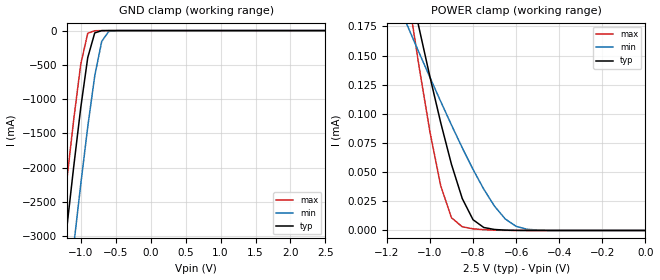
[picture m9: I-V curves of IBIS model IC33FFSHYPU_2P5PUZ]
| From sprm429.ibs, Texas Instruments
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|   Model IC33FFSHYPU_2P5PUZ
[Model]   IC33FFSHYPU_2P5PUZ
Model_type   Input
Polarity   Non-Inverting
Vinl =   0.7500V
Vinh =   1.7500V
C_comp   2.1510pF   2.1423pF   2.1675pF
[Temperature Range]   25.0000   0.1250k   -40.0000
[Voltage Range]   2.5000V   2.3000V   2.7000V
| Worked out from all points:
|   GND clamp passes 1 mA (typ) near -0.69 V on its own axis
|   POWER clamp passes 1 mA (typ) near -1.95 V on its own axis
[GND_clamp]
| voltage   I(typ)   I(min)   I(max)
-2.5V     -15.45A    -16.55A    -14.8A
-1.3V     -3.808A    -4.968A    -3.114A
-1.2V     -2.88A     -4.039A    -2.185A
-1.1V     -1.977A    -3.127A    -1.292A
-1V       -1.123A    -2.241A    -489.8mA
-900mV    -393.5mA   -1.402A    -39.29mA
-800mV    -34.07mA   -660.7mA   -2.405mA
-700mV    -1.067mA   -156.4mA   -232.2uA
-600mV    -42.99uA   -13.12mA   -13.27uA
-400mV    -95.57nA   -45.84uA   -11.77nA
2.5V      158.4pA    1.346nA    149.3pA
[POWER_clamp]
| voltage   I(typ)   I(min)   I(max)
-2.5V     1.522mA    806.3uA    2.102mA
-1.1V     216.2uA    173.8uA    200.1uA
-1.05V    173.4uA    152.4uA    140.2uA
-1V       131.9uA    131.4uA    84.68uA
-950mV    92.55uA    110.7uA    38.41uA
-900mV    56.73uA    90.48uA    10.93uA
-850mV    27.42uA    70.97uA    3.157uA
-800mV    9.238uA    52.44uA    1.436uA
-700mV    836.6nA    20.75uA    256.9nA
-600mV    104.4nA    3.55uA     18.68nA
-500mV    8.336nA    298nA      833.3pA
0V        158.4pA    1.104nA    166.9pA
